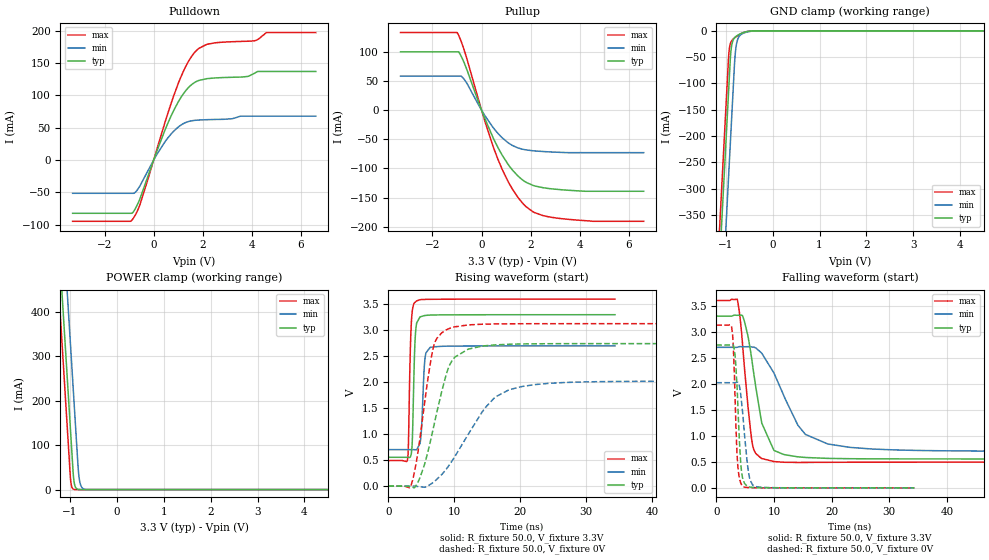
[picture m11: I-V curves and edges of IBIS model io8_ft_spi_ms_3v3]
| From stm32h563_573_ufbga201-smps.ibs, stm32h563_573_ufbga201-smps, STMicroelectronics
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[Model]   io8_ft_spi_ms_3v3
Model_type I/O
Polarity   Non-Inverting
Enable   Active-Low
| CAP_THRESHOLD on pad IOFT is "UDTCAPC" :
| Rising=20.0% of vddiom   Falling=80.0% of vddiom
| C_comp min and max val. don't necessarily correlate with the min and max pvt
| but are the smallest and greatest pad capacitance found.
| var   typ   min   max
C_comp   5.03682pF  4.97381pF  5.04445pF
|C_comp_pullup   3.26855pF  3.10790pF  3.04355pF
|C_comp_pulldown   1.76827pF  1.86591pF  2.00090pF
Vinl = 810.0mV
Vinh = 2.52V
Vmeas = 1.65V   | Reference voltage for timing measurements
Cref  = 50.0pF   | Timing specification test load capacitance value
Rref  = 100.0MOhm   | Timing specification test load resistance value
Vref  = 1.65V   | Timing specification test load voltage
[Model Spec]
| TIME_THRESHOLD on pin ZIV11 is "CMOS" :
| Rising=40.0% of vdd   Falling=60.0% of vdd
Vinl 1.29880V 1.07480V 1.40680V
Vinh 1.77520V 1.49320V 1.89720V
| variable   typ   min   max
[Temperature Range] 25.0 125.0 -40.0
| variable   typ   min   max
[Voltage Range] 3.3V 2.7V 3.6V
| variable   typ   min   max
[POWER Clamp Reference] 3.3V 2.7V 3.6V
| variable   typ   min   max
[GND Clamp Reference] 0V 0V 0V
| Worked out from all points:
|   slope of the pulldown table from 0 to 0.495 V, typ, clamps not added: 10 ohm
|   slope of the pullup table from 0 to 0.495 V, typ, clamps not added: 10 ohm
|   GND clamp passes 1 mA (typ) near -0.52 V on its own axis
|   POWER clamp passes 1 mA (typ) near -0.84 V on its own axis
|   rising waveform, R_fixture 50.0, V_fixture 3.3V: 20-80 % time 343ps typ, 427ps min, 330ps max; typ from 0.556 V to 3.3 V
|   falling waveform, R_fixture 50.0, V_fixture 3.3V: 20-80 % time 2.7ns typ, 5.42ns min, 1.54ns max; typ from 3.3 V to 0.556 V
|   rising waveform, R_fixture 50.0, V_fixture 0V: 20-80 % time 3.13ns typ, 6.25ns min, 2.1ns max; typ from 0 V to 2.74 V
|   falling waveform, R_fixture 50.0, V_fixture 0V: 20-80 % time 727ps typ, 1.05ns min, 589ps max; typ from 2.74 V to 0 V
[POWER Clamp]
-3.3V     4.068A     4.259A     3.957A
-1.25V    582.8mA    774.2mA    471.5mA
-1.13V    378.8mA    570.2mA    267.5mA
-1.09V    310.8mA    502.2mA    199.5mA
-1.02V    191.8mA    383.2mA    80.53mA
-990mV    140.8mA    332.2mA    29.53mA
-920mV    26.3mA     213.2mA    906uA
-880mV    5.543mA    145.2mA    123.7uA
-810mV    363.5uA    33.6mA     3.798uA
-770mV    76.62uA    10.47mA    519.4nA
-690mV    3.409uA    1.017mA    10.48nA
6.6V      0A         0A         0A
[GND Clamp]
-3.3V     -4.131A    -4.293A    -4.064A
-1.25V    -646.2mA   -808mA     -579.5mA
-940mV    -119.2mA   -281mA     -52.48mA
-920mV    -85.23mA   -247mA     -32.7mA
-900mV    -51.91mA   -213mA     -24.27mA
-870mV    -26.87mA   -162mA     -18.7mA
-810mV    -13.22mA   -60.41mA   -13.31mA
-790mV    -11.41mA   -38.37mA   -11.93mA
-740mV    -8.18mA    -15.37mA   -8.882mA
-660mV    -4.605mA   -6.274mA   -4.919mA
-320mV    -10.56uA   -77.76uA   -2.038uA
6.6V      9.514nA    1.879uA    704.5pA
| variable   typ   min   max
[Pullup Reference] 3.3V 2.7V 3.6V
| variable   typ   min   max
[Pulldown Reference] 0V 0V 0V
[Pullup]
-3.3V     100.3mA    58.58mA    133.4mA
-990mV    100.3mA    58.58mA    133.4mA
-910mV    98.91mA    58.58mA    126.4mA
-680mV    78.53mA    51.39mA    99.51mA
120mV     -12.96mA   -8.365mA   -16.99mA
680mV     -65.11mA   -40.43mA   -85.66mA
1.26V     -102.9mA   -60.65mA   -135.8mA
1.83V     -124.2mA   -68.3mA    -166.4mA
2.51V     -133.2mA   -71mA      -181.1mA
3.19V     -136.4mA   -72.38mA   -186mA
4.54V     -139.3mA   -72.9mA    -190.8mA
6.6V      -139.3mA   -72.9mA    -190.8mA
[Pulldown]
-3.3V     -82.43mA   -51.49mA   -94.82mA
-860mV    -81.66mA   -51.49mA   -91.78mA
-560mV    -60.16mA   -40.13mA   -69.41mA
120mV     12.61mA    7.999mA    15.37mA
800mV     75.3mA     43.94mA    97.52mA
1.33V     108.3mA    58.37mA    146.5mA
1.84V     123.1mA    61.83mA    172.7mA
2.51V     126.9mA    62.7mA     181.3mA
3.84V     129.3mA    67.77mA    183.7mA
4.13V     134.7mA    67.77mA    184.6mA
4.59V     136.9mA    67.77mA    197.1mA
6.6V      136.9mA    67.77mA    197.1mA
[Ramp]
dV/dt_r 1.64629V/3.12479ns 1.21235V/6.15122ns 1.87635V/2.101ns
dV/dt_f 1.64666V/2.37593ns 1.19801V/5.19881ns 1.86387V/1.54087ns
R_load = 50.0
| Removed startup time: 0s 0s 0s  .
| Removed end time: 34.4ns.
[Rising Waveform]
R_fixture   = 50.0
V_fixture   = 3.3V
V_fixture_min = 2.7V
V_fixture_max = 3.6V
0s        555.6mV    703.3mV    493.6mV
2.9ns     555.6mV    703.3mV    509.2mV
3.05ns    552.6mV    703.3mV    822.7mV
3.5ns     641.1mV    703.4mV    3.171V
4ns       2.656V     701.7mV    3.534V
4.3ns     3.142V     703.2mV    3.565V
4.95ns    3.264V     961.9mV    3.591V
5.6ns     3.286V     2.495V     3.594V
6.35ns    3.293V     2.672V     3.596V
34.4ns    3.3V       2.7V       3.6V
| Removed startup time: 0s 0s 0s  .
| Removed end time: 189.4ns.
[Falling Waveform]
R_fixture   = 50.0
V_fixture   = 3.3V
V_fixture_min = 2.7V
V_fixture_max = 3.6V
0s        3.3V       2.7V       3.6V
3.6ns     3.316V     2.7V       3.626V
4.6ns     3.296V     2.711V     2.701V
5.5ns     2.918V     2.713V     1.561V
6.4ns     2.278V     2.704V     775.3mV
7.9ns     1.242V     2.585V     563.7mV
10ns      719.8mV    2.207V     505.5mV
15.45ns   583.8mV    1.028V     488.8mV
23.2ns    560.2mV    777.7mV    492.5mV
189.4ns   555.6mV    703.3mV    493.6mV
| Removed startup time: 0s 0s 0s  .
| Removed end time: 99.3ns.
[Rising Waveform]
R_fixture   = 50.0
V_fixture   = 0V
V_fixture_min = 0V
V_fixture_max = 0V
0s        103.7nV    446.5nV    93.93nV
3.4ns     -16.18mV   31.4uV     1.841mV
4.9ns     201.3mV    -13.54mV   1.022V
6.1ns     712.6mV    14.1mV     2.145V
6.9ns     1.159V     81.36mV    2.705V
8.9ns     2.195V     346.3mV    3.015V
10.1ns    2.484V     571.7mV    3.067V
16.2ns    2.719V     1.714V     3.123V
22.3ns    2.74V      1.956V     3.127V
99.3ns    2.744V     2.021V     3.127V
| Removed startup time: 0s 0s 0s  .
| Removed end time: 34.35ns.
[Falling Waveform]
R_fixture   = 50.0
V_fixture   = 0V
V_fixture_min = 0V
V_fixture_max = 0V
0s        2.744V     2.021V     3.127V
2.7ns     2.747V     2.021V     3.06V
2.95ns    2.741V     2.021V     2.726V
3.25ns    2.549V     2.021V     1.77V
3.7ns     1.702V     2.029V     473.8mV
4.2ns     547.1mV    1.827V     109.3mV
4.6ns     173.1mV    1.414V     27.49mV
5.7ns     18.07mV    230.7mV    5.047mV
7ns       4.942mV    20.74mV    2.102mV
34.35ns   12.23uV    80.35uV    2.393uV
